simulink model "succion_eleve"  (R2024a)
settings: Solver=VariableStepAuto  StartTime=0.0  StopTime=10.0  RelTol=1e-3
libraries: fl_lib x11, nesl_utility x4, sh_lib x2, batteryecm_lib x1

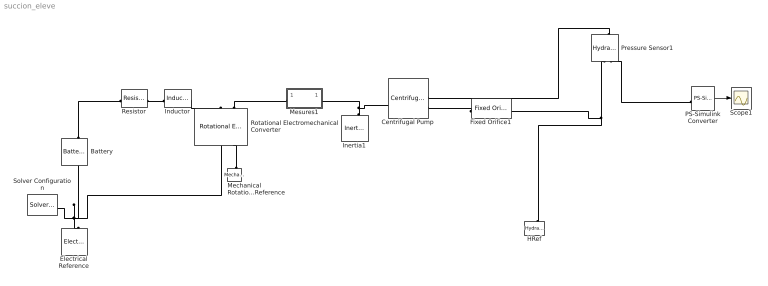
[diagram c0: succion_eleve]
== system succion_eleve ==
  Battery : batteryecm_lib/Battery  Vnom=12 V  prm_dir=simscape.enum.battery.prm_dir.disabled  R1_dis=2 Ohm  R1_ch=2 Ohm  R1=2 Ohm  prm_AH=simscape.enum.battery.prm_AH.infinite  AH=50 A*hr  V1=11.5 V  AH1=25 A*hr  prm_R2=simscape.enum.battery.prm_R2.disabled  R2=2000 Ohm  Tmeas=298.15 K  charge_measurement_port=simscape.enum.battery.enable.no  prm_dyn=simscape.enum.battery.prm_dyn.off  Rp1=0.005 Ohm  tau1=30 s  Rp2=0.005 Ohm  tau2=30 s  Rp3=0.005 Ohm  tau3=30 s  Rp4=0.005 Ohm  tau4=30 s  Rp5=0.005 Ohm  tau5=30 s  prm_fade=simscape.enum.battery.prm_fade.disabled  N_fade=100  AH_fade=45 A*hr  R1_fade=2.02 Ohm  R1_ch_fade=2.02 Ohm  V1_fade=10.35 V  prm_age=simscape.enum.battery.prm_age.disabled  prm_age_OCV=simscape.enum.battery.prm_age_OCV.OCV  OCV_age=0.9  SOC_age=60  Tmeas_age=298.15 K  delta_time_age_vec=[0] d  temperature_age_vec=[273] K  OCV_scaling_age=2.2134e6  OCV_offset_age=1.632e6  temp_exp_age=0.515833569 V  t_exp_age=0.75  Vnom_T2=12 V  R1_T2=2.2 Ohm  R1_T2_dis=2.2 Ohm  R1_T2_ch=2.2 Ohm  V1_T2=11.4 V  R2_T2=2200 Ohm  Rp1_T2=0.005 Ohm  tau1_T2=30 s  Rp2_T2=0.005 Ohm  tau2_T2=30 s  Rp3_T2=0.005 Ohm  tau3_T2=30 s  Rp4_T2=0.005 Ohm  tau4_T2=30 s  Rp5_T2=0.005 Ohm  tau5_T2=30 s  Tmeas2=273.15 K  thermal_port=simscape.enum.thermaleffects.omit  thermal_mass=30000 J/K  i_specify=off  i_priority=None  i=0 A  i_nominal_specify=off  i_nominal_value=1  i_nominal_unit=A  v_specify=off  v_priority=None  v=0 V  v_nominal_specify=off  v_nominal_value=1  v_nominal_unit=V  charge_specify=off  charge_priority=High  charge=50 A*hr  charge_nominal_specify=off  charge_nominal_value=1  charge_nominal_unit=A*hr  num_cycles_specify=off  num_cycles_priority=High  num_cycles=0  num_cycles_nominal_specify=off  num_cycles_nominal_value=1  num_cycles_nominal_unit=1  temperature_specify=off  temperature_priority=High  temperature=298.15 K  temperature_nominal_specify=off  temperature_nominal_value=1  temperature_nominal_unit=K
  Centrifugal Pump : sh_lib/Pumps and Motors/Centrifugal Pump  mdl_type=2  c_1=326.8 Pa/(kg/m^3)  c_2=3.104e+4 Pa*s/kg  c_3=1.097e+7 Pa*s^2/(kg*m^3)  c_4=2.136e+5 Pa*s^2/(kg*m^3)  c_f=0.8  design_del=130 lpm  ref_velocity=1.77e+3 rpm  ref_density=940 kg/m^3  leak_resistance=1e+8 Pa/(m^3/s)  T_const=0.1 N*m  trq_press_coeff=1e-6 N*m/Pa  pump_del_1D="[ 0  20.0   64.2   92.8  110.0  130.0] gpm"  press_diff_1D=[50.97 47.08 39.12 31.39 23.6 15.69] psi  pump_del_power_1D="[ 0  20.0   64.2   92.8  110.0  130.0] gpm"  power_1D="[0 7.8e-01   2.1   2.4   2.16   1.7] HP_DIN"  pump_vel_2D=[ 3.2e+3 3.3e+3 3.4e+3 3.5e+3 ] rpm  pump_del_2D=[ 0 50 100 150 200 250 300 350 ] lpm  press_diff_2D=[ 8.3 8.8 9.3 9.9; 7.8 8.3 8.8 9.4; 7.2 7.6 8.2 8.7; 6.5 7 7.5 8; 5.6 6.1 6.6 7.1; 4.7 5.2 5.7 6.2; 3.4 4 4.4 4.9; 2.3 2.7 3.4 3.6 ] bar  pump_del_power_2D=[ 0 50 100 150 200 250 300 350 ] lpm  power_2D=[ 1.223e+3 1.341e+3 1.467e+3 1.6e+3; 1.414e+3 1.551e+3 1.696e+3 1.85e+3; 1.636e+3 1.794e+3 1.962e+3 2.14e+3; 1.941e+3 2.129e+3 2.326e+3 2.54e+3; 2.224e+3 2.439e+3 2.66e+3 2.91e+3; 2.453e+3 2.691e+3 2.947e+3 3.21e+3; 2.757e+3 3.024e+3 3.307e+3 3.608e+3; 2.945e+3 3.23e+3 3.533e+3 3.854e+3 ] W  omega_threshold=1e-9 rad/s  interp_method=3  extrap_method=1
  Electrical Reference : fl_lib/Electrical/Electrical Elements/Electrical Reference
  Fixed Orifice1 : sh_lib/Orifices/Fixed Orifice  area=0.0001 m^2  C_d=0.7  lam_spec=1  B_lam=0.999  Re_cr=12  q_specify=off  q_priority=None  q=0.001 m^3/s  q_nominal_specify=off  q_nominal_value=1  q_nominal_unit=m^3/s  p_specify=off  p_priority=None  p=0 Pa  p_nominal_specify=off  p_nominal_value=1  p_nominal_unit=Pa
  HRef : fl_lib/Hydraulic/Hydraulic Elements/Hydraulic Reference
  Inductor : fl_lib/Electrical/Electrical Elements/Inductor  l=0.002 H  r=0 Ohm  g=1e-9 1/Ohm  i_specify=off  i_priority=High  i=0 A  i_nominal_specify=off  i_nominal_value=1  i_nominal_unit=A  v_specify=off  v_priority=High  v=0 V  v_nominal_specify=off  v_nominal_value=1  v_nominal_unit=V  i_L_specify=on  i_L_priority=High  i_L=0 A  i_L_nominal_specify=off  i_L_nominal_value=1  i_L_nominal_unit=A
  Inertia1 : fl_lib/Mechanical/Rotational Elements/Inertia  inertia=0.00002 kg*m^2  num_ports=foundation.enum.numPorts2.one  w_specify=on  w_priority=High  w=0 rad/s  w_nominal_specify=off  w_nominal_value=1  w_nominal_unit=rad/s  t_specify=off  t_priority=High  t=0 N*m  t_nominal_specify=off  t_nominal_value=1  t_nominal_unit=N*m
  Mechanical Rotational Reference : fl_lib/Mechanical/Rotational Elements/Mechanical Rotational Reference
  Mesures1 : Subsystem
  PS-Simulink Converter : nesl_utility/PS-Simulink Converter  PhysicalDomain=network_engine_domain  SubClassName=ps_output  LeftPortType=input  RightPortType=output  PseudoPeriodic=off  Frequencies=[]  VectorFormat=1-D array  Unit=atm  AffineConversion=off
  Pressure Sensor1 : fl_lib/Hydraulic/Hydraulic Sensors/Hydraulic Pressure Sensor
  Resistor : fl_lib/Electrical/Electrical Elements/Resistor  R=1 Ohm  i_specify=off  i_priority=High  i=0 A  i_nominal_specify=off  i_nominal_value=1  i_nominal_unit=A  v_specify=off  v_priority=High  v=0 V  v_nominal_specify=off  v_nominal_value=1  v_nominal_unit=V
  Rotational Electromechanical Converter : fl_lib/Electrical/Electrical Elements/Rotational Electromechanical Converter  K=0.2 V/(rad/s)  i_specify=off  i_priority=High  i=0 A  i_nominal_specify=off  i_nominal_value=1  i_nominal_unit=A  v_specify=off  v_priority=High  v=0 V  v_nominal_specify=off  v_nominal_value=1  v_nominal_unit=V  t_specify=off  t_priority=High  t=0 N*m  t_nominal_specify=off  t_nominal_value=1  t_nominal_unit=N*m  w_specify=off  w_priority=High  w=0 rad/s  w_nominal_specify=off  w_nominal_value=1  w_nominal_unit=rad/s
  Scope1 : Scope
  Solver Configuration : nesl_utility/Solver Configuration  PhysicalDomain=network_engine_domain  SubClassName=solver  LeftPortType=input  RightPortType=generic  Tones=[]  Harmonics=[]  SimulateNoise=off  Profile=off  UseLocalSampling=off  EnableSwitchedLinearOptims=on  FrequencyDomain=off  UseCCode=off  RelTol=0.001  AbsTol=1e-06  MinStep=1e-09  ToWorkspace=off  RevertToSquareIcSolve=off  NumHomotopyIterations=100  PhasorMode=off  PhasorModeNumHarmonics=1  ConsistencySolver=NEWTON_FTOL  IndexReductionMethod=DerivativeReplacement  DoDC=off  ResidualTolerance=1e-9  ConsistencyTolSource=GLOBAL  ConsistencyAbsTol=0.001  ConsistencyRelTol=0.001  ConsistencyTolFactor=0.001  UseLocalSolver=off  LocalSolverChoice=NE_BACKWARD_EULER_ADVANCER  ResolveIndetEquations=on  FunctionEvalNumThread=1  LocalSolverSampleTime=.001  DoFixedCost=off  MaxNonlinIter=3  MaxModeIter=2  ComputeImpulses=off  ImpulseIterations=2  LinearAlgebra=Sparse  LinearAlgebraNumThread=0  EquationFormulation=NE_TIME_EF  DelaysMemoryBudget=1024  AutomaticFiltering=on  FilteringTimeConstant=0.001  PartitionStorageMethod=AS_NEEDED  PartitionMemoryBudget=1024  PartitionMethod=FAST  MultibodyUseLocalSolver=off  MultibodyLocalSolverChoice=ODE1  MultibodyLocalSolverSampleTime=0.001
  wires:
  PS-Simulink Converter/1 -> Scope1/1
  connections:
  Electrical Reference/LConn1 -- Solver Configuration/RConn1 -- Rotational Electromechanical Converter/RConn1 -- Battery/RConn1
  Inertia1/LConn1 -- Centrifugal Pump/LConn1 -- Mesures1/RConn1
  Mechanical Rotational Reference/LConn1 -- Rotational Electromechanical Converter/RConn2
  Rotational Electromechanical Converter/LConn2 -- Mesures1/LConn1
  Resistor/RConn1 -- Inductor/LConn1
  Inductor/RConn1 -- Rotational Electromechanical Converter/LConn1
  Battery/LConn1 -- Resistor/LConn1
  Pressure Sensor1/LConn1 -- Centrifugal Pump/RConn1
  Fixed Orifice1/LConn1 -- Centrifugal Pump/RConn2
  PS-Simulink Converter/LConn1 -- Pressure Sensor1/RConn2
  HRef/LConn1 -- Fixed Orifice1/RConn1 -- Pressure Sensor1/RConn1

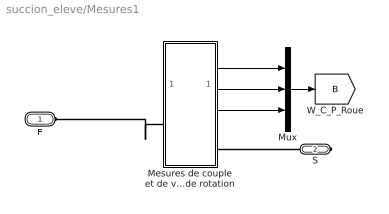
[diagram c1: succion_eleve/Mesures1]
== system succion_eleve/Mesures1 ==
  Mesures de couple et de vitesse de rotation : Subsystem
  Mux : Mux  Inputs=3
  E : PMIOPort  Side=Left
  S : PMIOPort  Port=2  Side=Right
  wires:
  Mesures de couple et de vitesse de rotation/3(Puissance) -> Mux/3
  Mux/1 -> [B]
  Mesures de couple et de vitesse de rotation/1(Vitesse) -> Mux/1
  Mesures de couple et de vitesse de rotation/2(Couple) -> Mux/2
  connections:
  Mesures de couple et de vitesse de rotation/LConn1 -- E/RConn1
  Mesures de couple et de vitesse de rotation/RConn1 -- S/RConn1

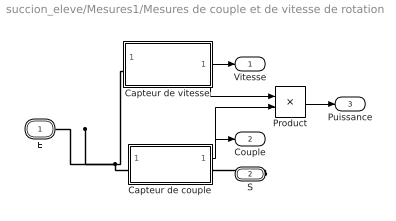
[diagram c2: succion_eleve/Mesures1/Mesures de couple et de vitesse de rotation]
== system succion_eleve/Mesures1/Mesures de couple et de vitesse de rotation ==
  Capteur de couple : Subsystem
  Capteur de vitesse : Subsystem
  Product : Product  RndMeth=Zero
  E : PMIOPort  Side=Left
  S : PMIOPort  Port=2  Side=Right
  Vitesse : Outport
  Couple : Outport  Port=2
  Puissance : Outport  Port=3
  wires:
  Product/1 -> Puissance/1
  Capteur de couple/1(Out1) -> Product/2, Couple/1
  Capteur de vitesse/1(Out1) -> Vitesse/1, Product/1
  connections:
  Capteur de couple/LConn1 -- Capteur de vitesse/LConn1 -- E/RConn1
  S/RConn1 -- Capteur de couple/RConn1

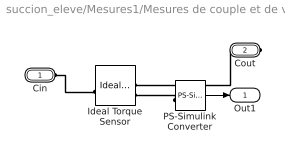
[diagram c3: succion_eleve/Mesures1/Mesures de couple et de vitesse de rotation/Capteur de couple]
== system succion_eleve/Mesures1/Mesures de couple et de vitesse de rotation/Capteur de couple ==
  Ideal Torque Sensor : fl_lib/Mechanical/Mechanical Sensors/Ideal Torque Sensor
  PS-Simulink Converter : nesl_utility/PS-Simulink Converter  PhysicalDomain=network_engine_domain  SubClassName=ps_output  LeftPortType=input  RightPortType=output  PseudoPeriodic=off  Frequencies=[]  VectorFormat=1-D array  Unit=1  AffineConversion=off
  Cin : PMIOPort  Side=Left
  Cout : PMIOPort  Port=2  Side=Right
  Out1 : Outport
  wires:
  PS-Simulink Converter/1 -> Out1/1
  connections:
  Cout/RConn1 -- Ideal Torque Sensor/RConn1
  PS-Simulink Converter/LConn1 -- Ideal Torque Sensor/RConn2
  Cin/RConn1 -- Ideal Torque Sensor/LConn1

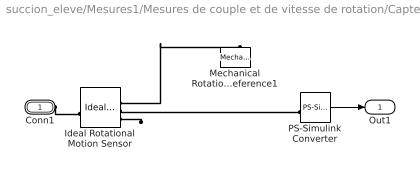
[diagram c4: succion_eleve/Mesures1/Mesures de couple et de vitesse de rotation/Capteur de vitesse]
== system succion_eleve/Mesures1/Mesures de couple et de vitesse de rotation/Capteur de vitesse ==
  Ideal Rotational Motion Sensor : fl_lib/Mechanical/Mechanical Sensors/Ideal Rotational Motion Sensor  reference=foundation.enum.MeasurementReference.difference  acceleration_port=false  velocity_port=true  position_port=true  wrap_angle=false  offset=0 rad
  Mechanical Rotational Reference1 : fl_lib/Mechanical/Rotational Elements/Mechanical Rotational Reference
  PS-Simulink Converter : nesl_utility/PS-Simulink Converter  PhysicalDomain=network_engine_domain  SubClassName=ps_output  LeftPortType=input  RightPortType=output  PseudoPeriodic=off  Frequencies=[]  VectorFormat=1-D array  Unit=1  AffineConversion=off
  Conn1 : PMIOPort  Side=Left
  Out1 : Outport
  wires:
  PS-Simulink Converter/1 -> Out1/1
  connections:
  Ideal Rotational Motion Sensor/RConn3 -- ?
  Conn1/RConn1 -- Ideal Rotational Motion Sensor/LConn1
  Ideal Rotational Motion Sensor/RConn2 -- PS-Simulink Converter/LConn1
  Ideal Rotational Motion Sensor/RConn1 -- Mechanical Rotational Reference1/LConn1
